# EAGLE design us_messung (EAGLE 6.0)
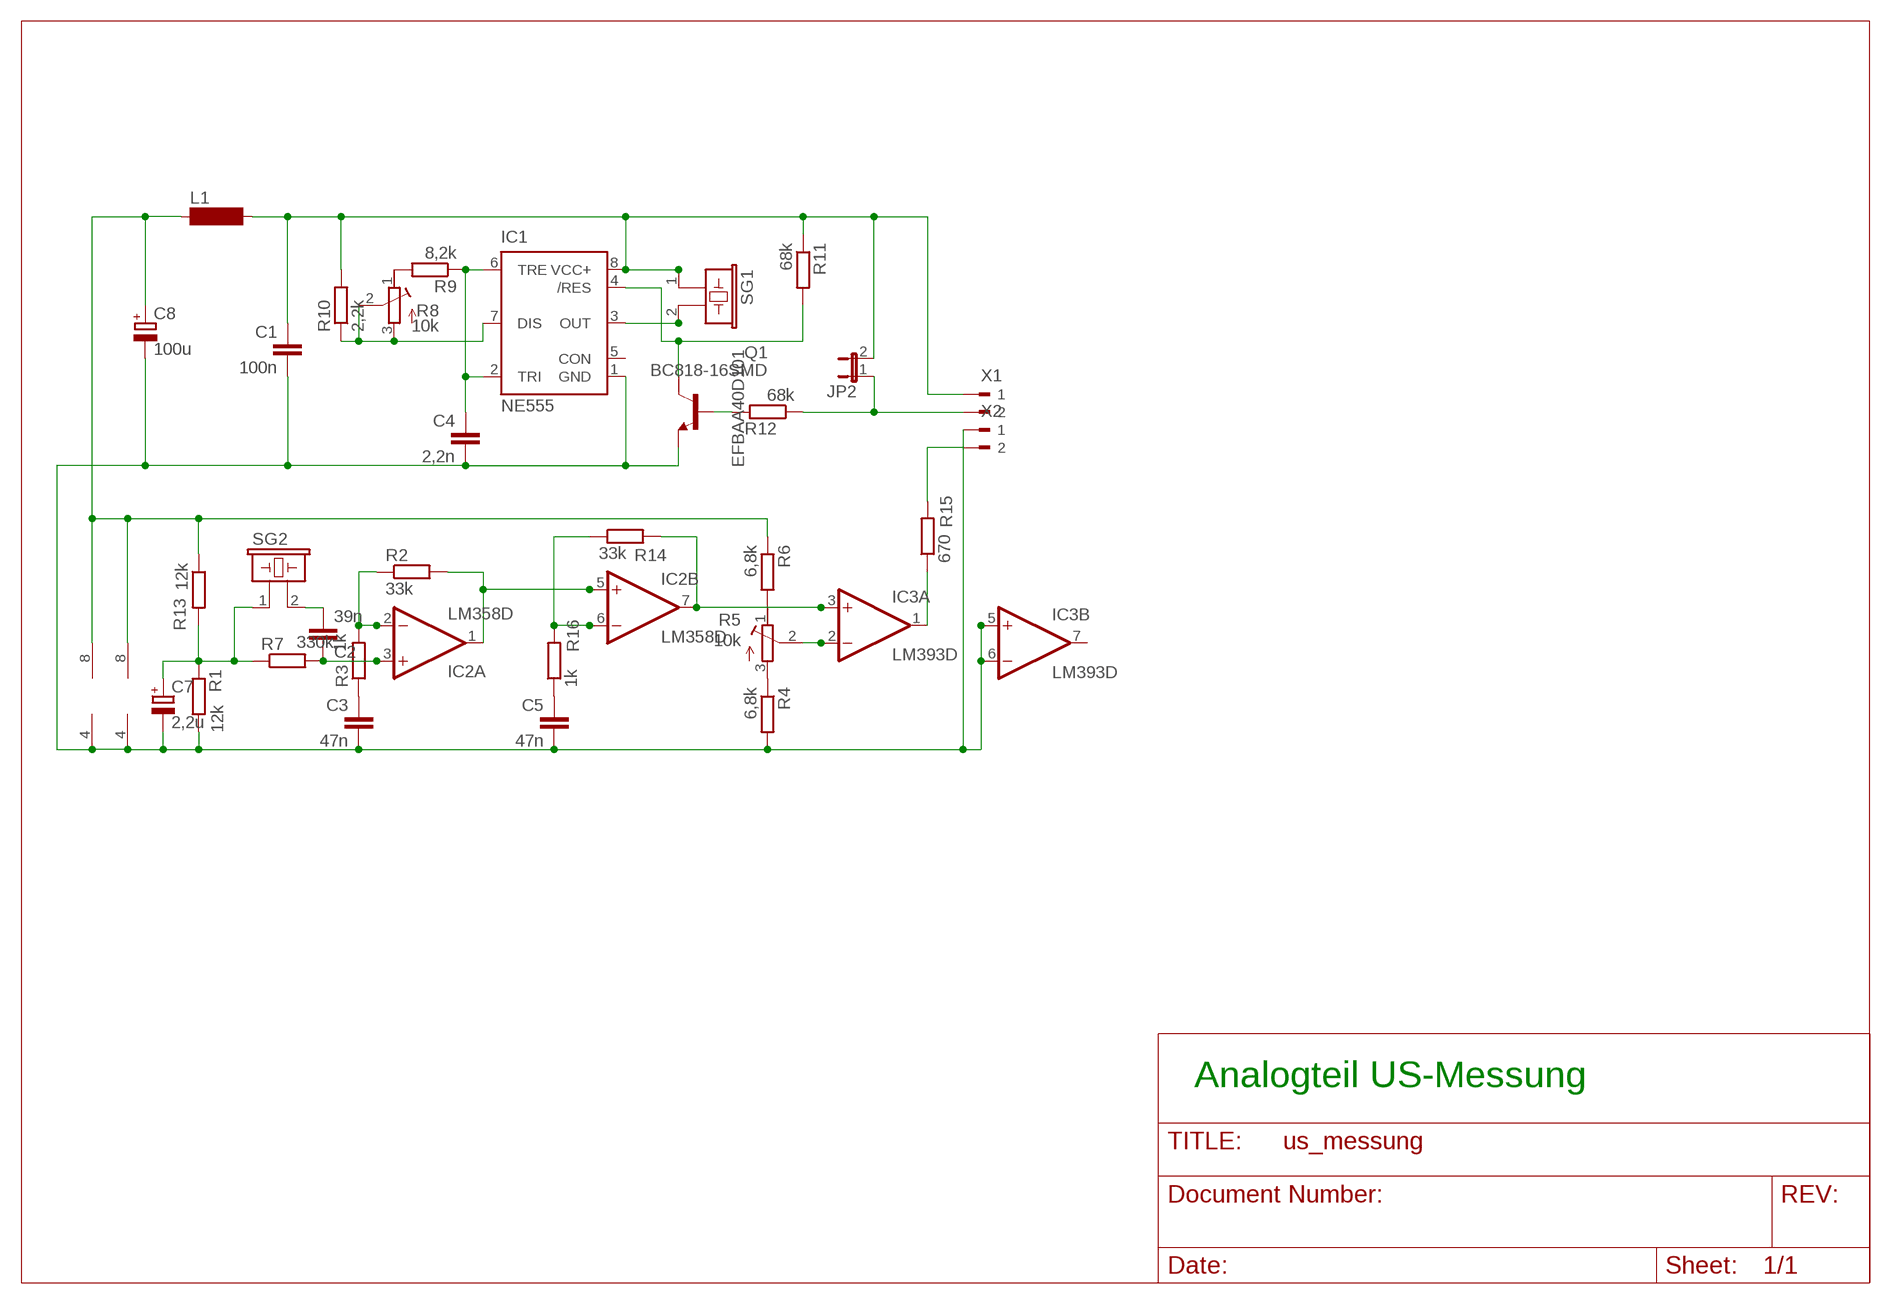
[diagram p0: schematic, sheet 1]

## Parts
C1  100n  C-EUC0805  [C0805]
C2  39n  C-EUC0805  [C0805]
C3  47n  C-EUC0805  [C0805]
C4  2,2n  C-EUC0805  [C0805]
C5  47n  C-EUC0805  [C0805]
C7  2,2u  CPOL-EUC/6032-28R  [C/6032-28R]
C8  100u  CPOL-EU153CLV-0605  [153CLV-0605]
IC1  NE555  [SO08]
IC2  LM358D  [SO08]
IC3  LM393D  [SO08]
JP2  JP1E  [JP1]
L1  SM-NE45  [SM-NE45]
Q1  BC818-16SMD  [SOT23-BEC]
R1  12k  R-EU_R1206  [R1206]
R2  33k  R-EU_R1206  [R1206]
R3  1k  R-EU_R1206  [R1206]
R4  6,8k  R-EU_R1206  [R1206]
R5  10k  R-TRIMMT93YA  [RTRIMT93YA]
R6  6,8k  R-EU_R1206  [R1206]
R7  330k  R-EU_R1206  [R1206]
R8  10k  R-TRIMMT93YA  [RTRIMT93YA]
R9  8,2k  R-EU_R1206  [R1206]
R10  2,2k  R-EU_R1206  [R1206]
R11  68k  R-EU_R1206  [R1206]
R12  68k  R-EU_R1206  [R1206]
R13  12k  R-EU_R1206  [R1206]
R14  33k  R-EU_R1206  [R1206]
R15  670  R-EU_R1206  [R1206]
R16  1k  R-EU_R1206  [R1206]
SG1  EFBAA40D101  [EFBAA40D101]
SG2  EFBAA40D101  [EFBAA40D101]
X1  90-290-2_CLAMP  [CLAMP]
X2  90-290-2_CLAMP  [CLAMP]

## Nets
GND: C1.2 C3.2 C4.2 C5.2 C7.- C8.- IC1.1(GND) IC2.4(P:V-) IC3.4(P:V-) IC3.5(B:+IN) IC3.6(B:-IN) Q1.E R1.2 R4.2 X2.P$1
N$1: IC3.1(A:OUT) R15.1
N$2: C2.2 SG2.2
N$3: C3.1 R3.1
N$4: IC1.4(/RES) Q1.C R11.2
N$5: C2.1 IC2.3(A:+IN) R7.2
N$6: IC1.3(OUT) SG1.2
N$7: Q1.B R12.2
N$8: C7.+ R1.1 R7.1 R13.2 SG2.1
N$9: C4.1 IC1.2(TRI) IC1.6(TRE) R9.1
N$10: IC2.1(A:OUT) IC2.5(B:+IN) R2.2
N$11: IC2.2(A:-IN) R2.1 R3.2
N$12: C5.1 R16.1
N$13: R8.1(A) R9.2
N$14: IC2.6(B:-IN) R14.1 R16.2
N$15: IC2.7(B:OUT) IC3.3(A:+IN) R14.2
N$16: IC1.7(DIS) R8.2(S) R8.3(E) R10.1
N$17: R4.1 R5.3(E)
N$18: R5.1(A) R6.2
N$19: R15.2 X2.P$2
N$20: JP2.1 R12.1 X1.P$2
N$21: IC3.2(A:-IN) R5.2(S)
V5: C8.+ IC2.8(P:V+) IC3.8(P:V+) L1.1 R6.1 R13.1
V12: C1.1 IC1.8(VCC+) JP2.2 L1.2 R10.2 R11.1 SG1.1 X1.P$1
Unconnected: IC1.5(CON) IC3.7(B:OUT)

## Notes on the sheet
- Analogteil US-Messung

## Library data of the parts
C1-C5 = resistor:C-EU: CAPACITOR, European symbol
C7 C8 = resistor:CPOL-EU: POLARIZED CAPACITOR, European symbol
IC1 = st-microelectronics:NE555: General purpose bipolar Timer
IC2 = linear:LM358: OP AMP also LM158; LM258; LM2904 Source: http://cache.national.com/ds/LM/LM158.pdf
IC3 = linear:LM393: COMPARATOR
JP2 = jumper:JP1E: JUMPER
L1 = Mylib:SM-NE45: INDUCTOR; OC_FARNELL: unknown; OC_NEWARK: unknown
Q1 = Mylib:BC818*: NPN Transistor
R1-R4 R6 R7 R9-R16 = resistor:R-EU_: RESISTOR, European symbol
R5 R8 = resistor:R-TRIMM: Trimm resistor
SG1 SG2 = buzzer:EFB?: Piezoelectric Acoustic Transducer; OC_FARNELL: unknown; OC_NEWARK: unknown
X1 X2 = Mylib:90-2: WEIDMUELLER CLAMP CONNECTOR

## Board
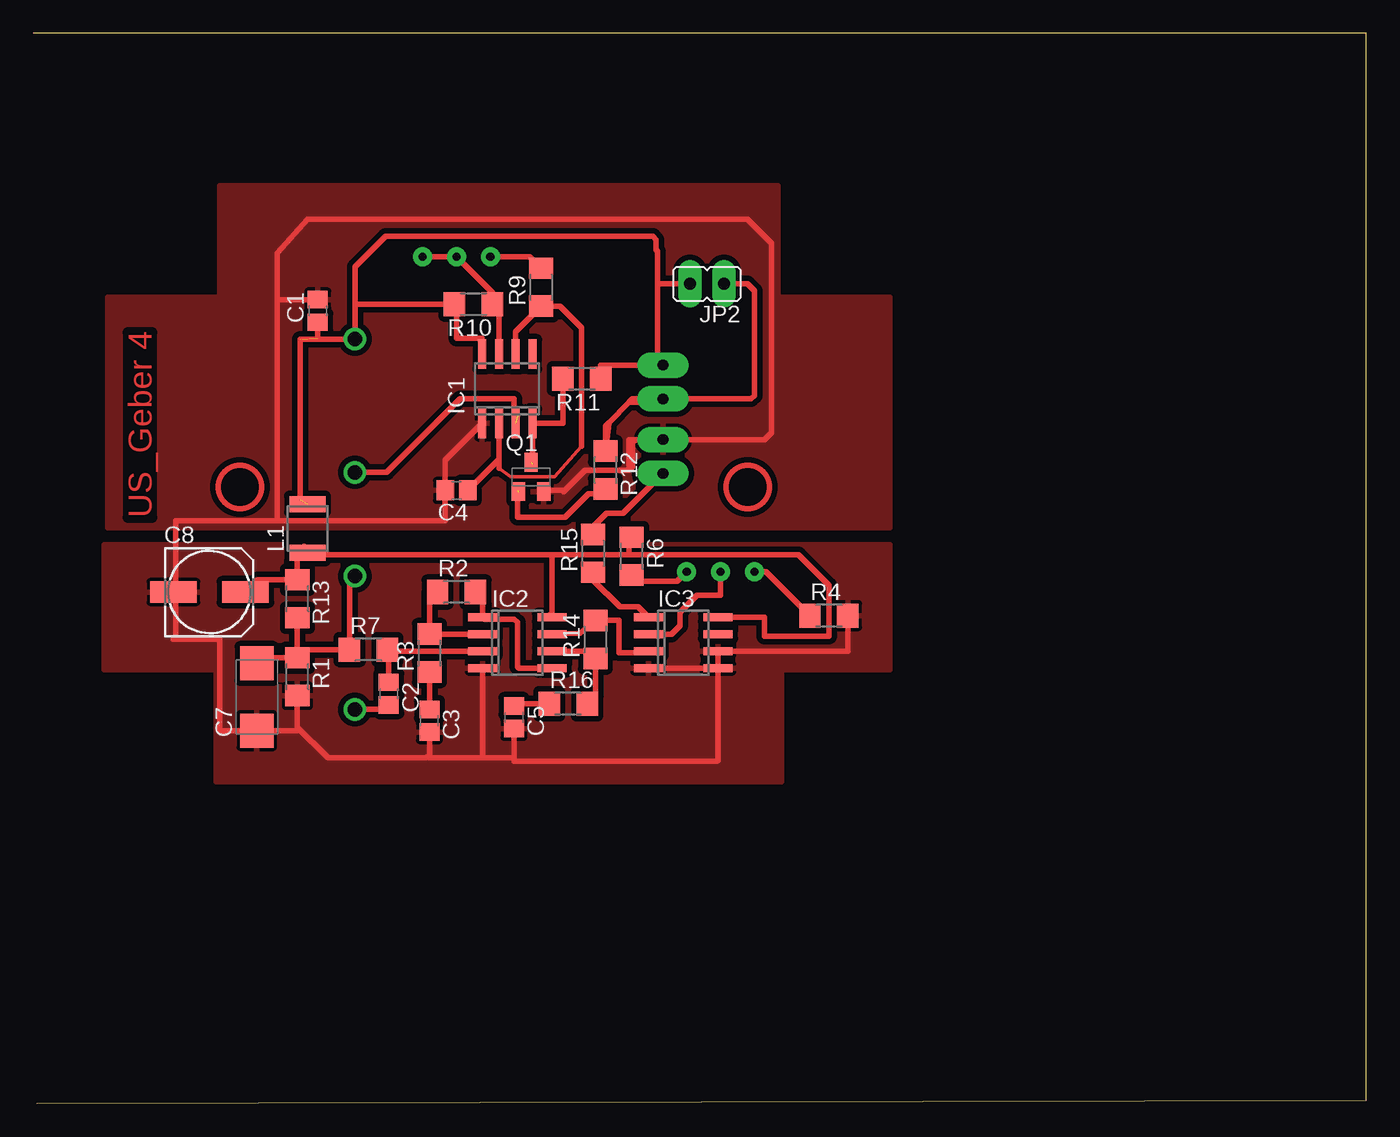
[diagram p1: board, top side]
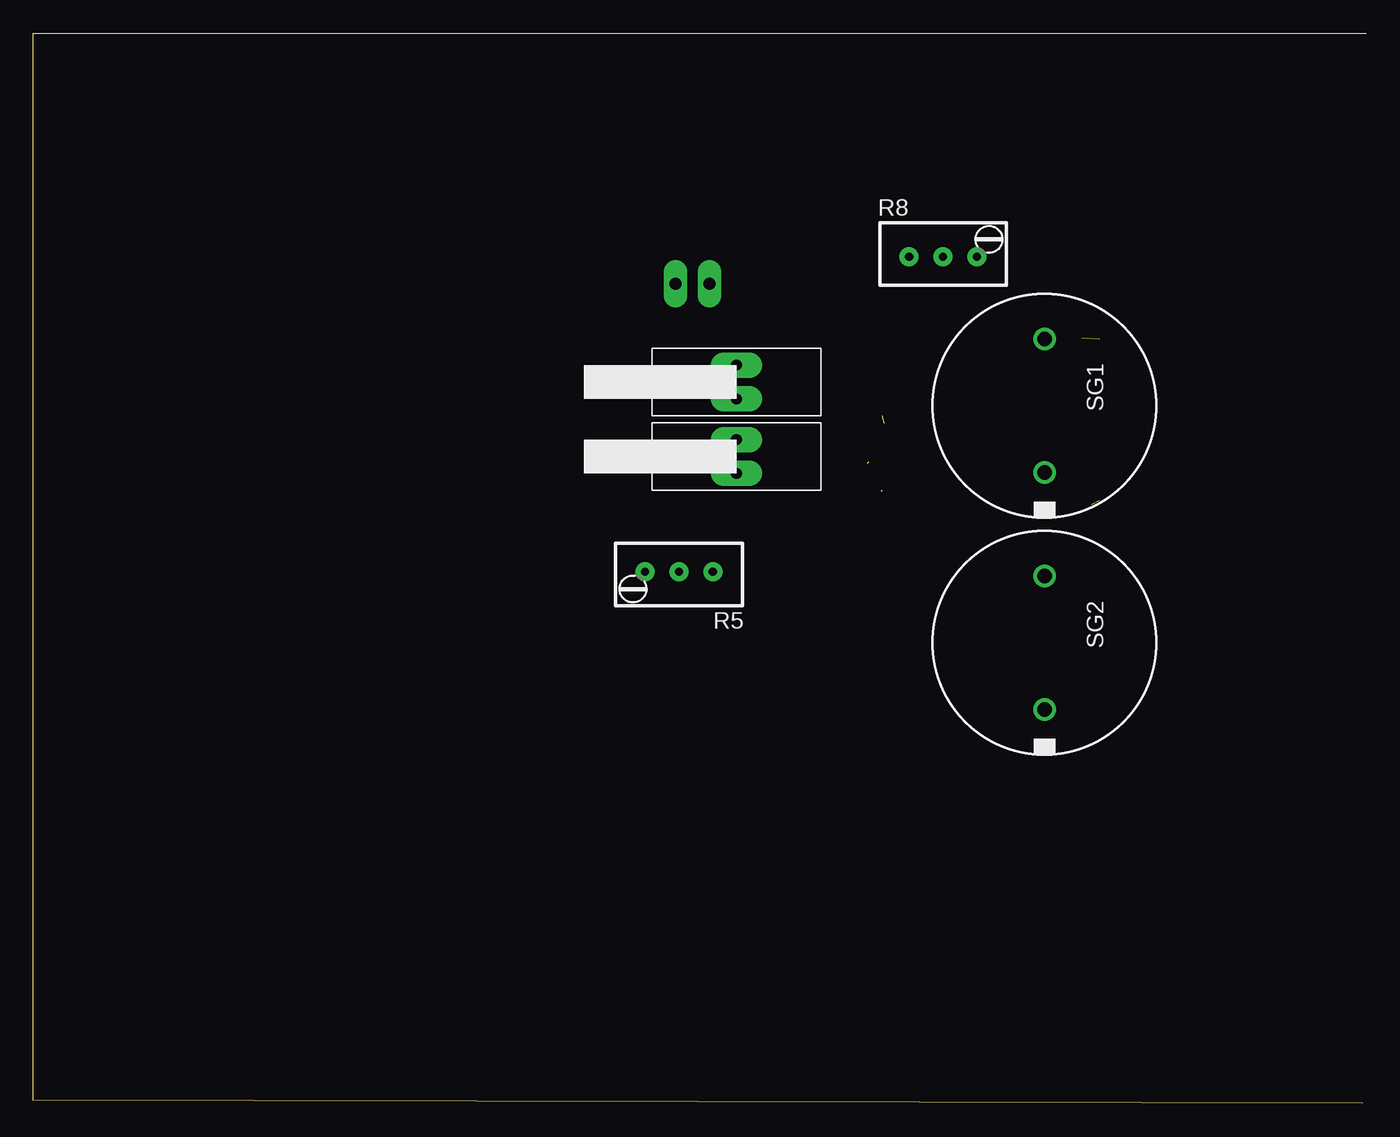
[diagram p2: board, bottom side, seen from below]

Size 100 x 80.25 mm. Coordinates in mm from the lower left corner, seen from the top.
Outline: 0.25,0 100,0.25 100,80.25 0,80.25
Copper layers (1*16): Top 0.035mm / dielectric 1.5mm / Bottom 0.035mm
Design rules: minimum track width 10mil, minimum drill 24mil, track to track 8mil, track to pad 8mil, pad to pad 8mil, via to via 8mil, smd to smd 8mil, copper to edge 40mil, drill to drill 8mil, minimum pad ring 10mil, minimum via ring 8mil, stop-mask expansion 4mil, vias tented up to drill 0mil, thermal gap 10mil

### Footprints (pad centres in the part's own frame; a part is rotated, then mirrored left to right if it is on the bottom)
C0805 = smd 1.3 x 1.5: 1 -0.85,0; 2 0.85,0
C/6032-28R = smd 2.55 x 2.5: + 2.525,0; - -2.525,0
153CLV-0605 = smd 3.5 x 1.6: + 2.7,0; - -2.7,0
SO08 = smd 0.6 x 2.2: 1 -1.905,-2.6; 2 -0.635,-2.6; 3 0.635,-2.6; 4 1.905,-2.6; 5 1.905,2.6; 6 0.635,2.6; 7 -0.635,2.6; 8 -1.905,2.6
JP1 = drill 0.914 pad 1.778 long: 1 0,-1.27; 2 0,1.27
SM-NE45 = smd 1.2 x 2.7: 1 -2.15,0; 2 1.515,0
SOT23-BEC = smd 1 x 1.4: B -0.95,-1.1; C 0,1.1; E 0.95,-1.1
R1206 = smd 1.6 x 1.803: 1 -1.422,0; 2 1.422,0
RTRIMT93YA = drill 0.61 pad 1.422: 1 0,-2.54; 2 0,0; 3 0,2.54
EFBAA40D101 = drill 1.1 pad 1.676: 1 -5,0; 2 5,0
CLAMP = drill 0.8 pad 1.93 long: P$1 -1.27,0; P$2 1.27,0

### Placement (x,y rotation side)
C1  21.34,59.44 90 top
C2  26.67,30.73 270 top
C3  29.72,28.7 270 top
C4  31.75,45.97 180 top
C5  36.07,28.96 270 top
C7  16.76,30.48 90 top
C8  13.21,38.35 0 top
IC1  35.56,53.59 0 top
IC2  36.32,34.54 270 top
IC3  48.77,34.54 270 top
JP2  50.55,61.47 90 top
L1  20.57,43.43 90 top
Q1  37.34,46.99 0 top
R1  19.81,32 270 top
R2  31.75,38.35 0 top
R3  29.72,33.78 90 top
R4  59.69,36.58 0 top
R5  51.56,39.88 90 bottom
R6  44.89,41.04 270 top
R7  25.15,34.04 0 top
R8  31.75,63.5 270 bottom
R9  38.1,61.21 90 top
R10  33.02,59.94 180 top
R11  41.15,54.36 180 top
R12  42.93,47.5 270 top
R13  19.81,37.85 270 top
R14  42.16,34.8 90 top
R15  42,41.25 90 top
R16  40.13,29.97 0 top
SG1  24.13,52.32 270 bottom
SG2  24.13,34.54 270 bottom
X1  47.24,54.1 270 bottom
X2  47.24,48.51 270 bottom

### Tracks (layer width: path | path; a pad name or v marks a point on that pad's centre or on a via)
GND
  Top 0.406: R1.2 19.81,30.23 | R1.2 19.81,28.21 22.11,25.91 29.46,25.91 29.72,26.16 C3.2 29.72,25.91 33.72,25.91 | IC3.5 IC3.6 61.11,33.91 R4.2 | IC3.5 IC3.4 | 36.07,25.91 C5.2 | IC3.5 51.31,32.64 | 33.78,25.91 33.72,25.97 IC2.4 33.72,25.91 | 39.88,45.97 39.79,45.89 | 44.7,47.5 44.96,47.75 44.96,49.53 45.21,49.78 X2.P$1 | C7.- 16.26,28.19 | IC1.1 30.9,48.24 C4.2 30.9,43.69 18.29,43.69 | 33.72,25.91 33.78,25.91 | 33.78,25.91 36.07,25.91 | 36.07,25.91 36.07,25.65 51.31,25.65 51.37,25.71 IC3.5 | C7.- 13.97,27.96 13.97,34.8 10.67,34.8 | 10.67,34.8 10.51,34.8 | C7.- 19.81,27.96 R1.2 | 10.67,34.8 10.67,38.19 C8.- 10.67,38.35 10.67,43.69 18.29,43.69 | 39.88,45.97 38.37,45.97 | 39.88,45.97 41.4,47.5 44.7,47.5 | 44.7,47.5 44.7,49.78 X2.P$1 | X2.P$1 54.86,49.78 55.37,50.29 55.37,64.52 53.59,66.29 20.57,66.29 18.29,63.75 18.29,60.29 | 18.29,43.69 18.29,60.2 18.29,60.29 | C1.2 18.29,60.29
  pour Top (isolate 0.406): 13.97,60.45 13.97,68.83 55.88,68.83 55.88,60.45 64.26,60.45 64.26,43.18 5.59,43.18 5.59,60.45
  pour Top (isolate 0.406): 5.33,32.51 5.33,41.91 64.26,41.91 64.26,32.51 56.13,32.51 56.13,24.13 13.72,24.13 13.72,32.51
N$1
  Top 0.406: R15.1 42,39.25 44,37.25 45.36,37.25 IC3.1
N$2
  Top 0.406: C2.2 26.33,29.54 SG2.2
N$3
  Top 0.406: C3.1 R3.1
N$4  (1 unrouted)
  Top 0.406: IC1.4 37.34,50.87 | IC1.4 39.73,50.99 R11.2 | 37.47,47.96 IC1.4
N$5
  Top 0.406: IC2.3 26.7,33.91 R7.2 26.67,33.93 C2.1
N$6  (1 unrouted)
  Top 0.406: SG1.2 26.5,47.32 32,52.83 36.07,52.83 36.07,51.82 36.32,51.56
N$7  (1 unrouted)
  Top 0.406: R12.2 42.57,45.72 41.66,45.72 39.88,43.94 36.32,43.94 36.32,45.97
N$8
  Top 0.406: C7.+ 16.42,33.43 R1.1 | R1.1 R13.2 | R1.1 19.81,34.04 R7.1 23.72,39.14 SG2.1
N$9
  Top 0.254: 34.92,47.62 35.81,46.99 39.12,46.99 41.15,49.28
  Top 0.406: IC1.6 36.2,57.89 R9.1 39.52,59.79 41.15,58.17 41.15,49.28 | C4.1 34.92,48.3 IC1.2 34.92,47.62
N$10
  Top 0.406: R2.2 33.72,38.35 IC2.1 33.85,36.32 36.07,36.32 36.32,36.07 36.32,32.77 36.45,32.64 IC2.5
N$11
  Top 0.406: R2.1 29.72,38.35 R3.2 33.72,35.2 IC2.2
N$12
  Top 0.406: C5.1 36.07,29.97 R16.1
N$13
  Top 0.406: R8.1 37.24,63.5 R9.2
N$14
  Top 0.406: IC2.6 41.63,33.91 arc-90 R14.1 42.16,30.58 R16.2
N$15
  Top 0.406: IC2.7 41,35.25 R14.2 43.94,36.22 43.94,33.78 46.17,33.78 IC3.3
N$16
  Top 0.406: R8.3 R8.2 34.44,60.81 R10.1 34.92,59.46 IC1.7
N$17
  Top 0.406: R4.1 54.97,39.88 R5.3
N$18
  Top 0.406: R6.2 45.37,39.15 48.29,39.15 R5.1
N$19
  Top 0.406: 47.29,47.2 X2.P$2 44.25,44.25 43,44.25 42,43.25 R15.2
N$20
  Top 0.406: 44.7,52.58 46.99,52.58 X1.P$2 | 43.18,51.05 42.93,50.8 R12.1 43.18,51.05 | 43.18,51.05 44.7,52.58 | 44.7,52.58 44.96,52.83 53.85,52.83 54.1,53.09 54.1,60.96 53.59,61.47 JP2.1
N$21
  Top 0.406: IC3.2 47.88,35.18 48.51,35.81 48.51,36.83 49.78,38.1 51.56,38.1 R5.2
V5
  Top 0.406: R13.1 20,39.46 | 38.73,36.64 IC2.8 38.92,41.15 | 38.92,41.15 44.7,41.15 | 44.7,41.15 44.7,42.46 R6.1 | R13.1 19.81,39.12 | C8.+ 16.82,39.27 R13.1 | 44.7,41.15 57.4,41.15 59.69,38.86 59.69,35.05 54.86,35.05 54.86,36.45 IC3.8 | 20.32,41.66 20.32,41.79 L1.1 20.57,41.15 | 38.92,41.15 20.57,41.15 | 20.57,41.15 19.81,41.15 R13.1
V12  (2 unrouted)
  Top 0.406: IC1.8 33.66,57.4 31.75,57.4 31.75,59.94 R10.2 24.13,59.94 | 24.13,59.94 SG1.1 20.02,57.32 | 46.82,61.47 46.82,55.37 X1.P$1 42.57,55.37 R11.1 | 46.82,61.47 46.82,63.92 46.74,64.01 46.74,64.77 46.48,65.02 26.42,65.02 24.13,62.74 24.13,59.94 | 46.82,61.47 JP2.2 | 20.02,57.32 20,57.31 | 20.02,45.22 20.02,57.32 | C1.1 21.34,57.4
(copper drawn outside any net)
  shapes: Top circle x2

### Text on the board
Top: US_Geber 4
